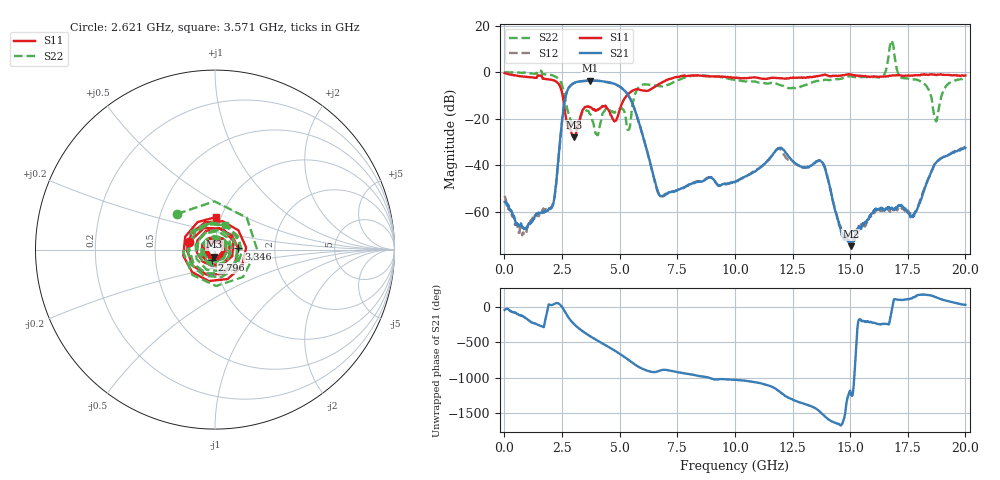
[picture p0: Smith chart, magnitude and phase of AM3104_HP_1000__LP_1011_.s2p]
!Created with skrf (http://scikit-rf.org).
# Hz S RI R 50.0
!freq ReS11 ImS11 ReS21 ImS21 ReS12 ImS12 ReS22 ImS22
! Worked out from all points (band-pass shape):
!   1601 points, 10 MHz to 20 GHz, reference 50 ohm
!   highest |S21| = -3.58 dB at 3.721 GHz (marker M1); lowest = -74.8 dB at 15.03 GHz (marker M2)
!   |S21| within 3 dB of the highest: 2.797 GHz to 5.061 GHz (2.265 GHz wide, 57.6 % of centre)
!   lowest |S11| = -28.0 dB at 3.009 GHz (marker M3), VSWR 1.08, Z = 49.4 - j3.91 ohm
!   |S11| at or under -10 dB: 2.528 GHz to 5.308 GHz (2.78 GHz wide, 71 % of centre)
!   |S22| runs from -27.1 to 13.6 dB; largest |S21 - S12| = 0.054
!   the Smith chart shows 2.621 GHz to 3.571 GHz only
!   S11 on the Smith chart (normalised r, x): 2.621 GHz: 0.75, +0.07; 2.796 GHz: 0.96, -0.11; 3.346 GHz: 1.30, +0.02; 3.571 GHz: 0.95, +0.36
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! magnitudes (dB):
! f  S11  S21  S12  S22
! 10 MHz  -0.4  -55.8  -53.2  0.0
! 834.6 MHz  -1.9  -67.3  -69.0  -0.2
! 2.021 GHz  -3.2  -58.6  -58.1  -1.2
! 2.621 GHz  -16.5  -12.2  -12.2  -10.8
! 2.796 GHz  -24.4  -6.6  -6.6  -18.3
! 3.009 GHz  -28.0  -4.7  -4.8  -23.5
! 3.346 GHz  -17.7  -3.9  -3.9  -18.0
! 3.571 GHz  -14.8  -3.7  -3.7  -16.6
! 3.721 GHz  -15.0  -3.6  -3.6  -18.1
! 4.795 GHz  -21.0  -5.1  -5.1  -17.4
! 5.395 GHz  -9.2  -10.3  -10.3  -24.7
! 5.795 GHz  -7.3  -20.3  -20.3  -6.9
! 6.682 GHz  -5.3  -51.9  -52.1  -5.9
! 10.01 GHz  -2.5  -47.3  -47.1  -3.4
! 11.92 GHz  -2.6  -32.6  -32.8  -5.4
! 13.34 GHz  -2.2  -40.0  -40.0  -4.4
! 13.84 GHz  -1.2  -39.9  -39.4  -3.5
! 15.03 GHz  -1.0  -74.8  -70.9  -1.8
! 16.68 GHz  -1.6  -58.4  -59.5  7.2
! 17.71 GHz  -1.5  -61.9  -62.3  -3.2
! 18.71 GHz  -1.2  -39.0  -39.1  -20.9
! 20 GHz  -1.4  -32.5  -32.2  -2.6
